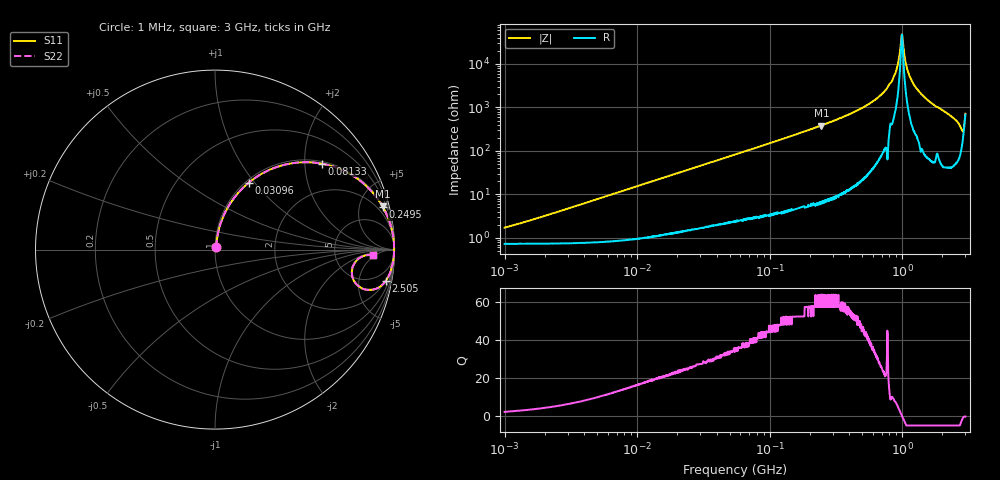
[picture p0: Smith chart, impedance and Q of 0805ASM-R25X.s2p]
!s-Parameter Generated by FASTRON Sdn. Bhd.
!FASTRON P/N : 0805ASM-R25X
!Keysight Technologies: E4991B_MY54100416_A.01.15
!Date: Fri Jun 19 14:51:25 2026
!Version  :Rev00  Fri Jun 19 14:51:25 2026
!Data & Calibration Information:
!Freq  S11  S21  S12  S22
!PortZ  Port1:50+j0  Port2:50+j0
!When reading reference impedance value at option line is always used.
! Remarks : This data is being provided solely for informational purposes.
# Hz S dB R 50
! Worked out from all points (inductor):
!   1601 points, 1 MHz to 3 GHz, reference 50 ohm
!   read as one part in series: L = 247 nH near 1.412 MHz
!   highest Q = 63.5 at 245.8 MHz (marker M1), where L = 249 nH
!   self-resonance near 992.8 MHz
!   S11 on the Smith chart (normalised r, x): 1 MHz: 1.01, +0.03; 30.96 MHz: 1.03, +0.94; 81.33 MHz: 1.06, +2.44; 249.5 MHz: 1.14, +7.87; 2.505 GHz: 2, -11; 3 GHz: 15, -4
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1000000  -35.40 64.0  -0.06 -0.9  -0.06 -0.9  -35.40 64.0
3804036  -24.60 79.3  -0.08 -3.3  -0.08 -3.3  -24.60 79.3
1.447069e7  -13.40 74.8  -0.30 -12.4  -0.30 -12.4  -13.40 74.8
3.096105e7  -7.56 63.2  -0.98 -24.7  -0.98 -24.7  -7.56 63.2
5.504702e7  -4.03 49.4  -2.39 -38.9  -2.39 -38.9  -4.03 49.4
8.132864e7  -2.33 38.8  -4.06 -49.8  -4.06 -49.8  -2.33 38.8
2.083556e8  -0.44 17.2  -10.60 -71.8  -10.60 -71.8  -0.44 17.2
2.457655e8  -0.32 14.5  -12.00 -74.6  -12.00 -74.6  -0.32 14.5
2.494827e8  -0.31 14.2  -12.20 -74.8  -12.20 -74.8  -0.31 14.2
5.337858e8  -0.05 5.2  -20.80 -83.5  -20.80 -83.5  -0.05 5.2
6.889699e8  -0.03 3.0  -25.70 -84.8  -25.70 -84.8  -0.03 3.0
7.925923e8  -0.02 1.8  -30.30 -84.8  -30.30 -84.8  -0.02 1.8
8.937307e8  -0.02 0.9  -36.20 -81.1  -36.20 -81.1  -0.02 0.9
9.730857e8  -0.02 0.2  -48.20 -57.4  -48.20 -57.4  -0.02 0.2
9.977393e8  -0.02 -0.0  -53.60 7.0  -53.60 7.0  -0.02 -0.0
1.023018e9  -0.02 -0.2  -47.30 60.9  -47.30 60.9  -0.02 -0.2
1.108292e9  -0.02 -0.9  -36.30 80.9  -36.30 80.9  -0.02 -0.9
1.255985e9  -0.03 -1.9  -29.50 83.5  -29.50 83.5  -0.03 -1.9
1.581072e9  -0.05 -4.0  -23.10 83.4  -23.10 83.4  -0.05 -4.0
2.505452e9  -0.29 -10.4  -14.80 74.3  -14.80 74.3  -0.29 -10.4
2.811057e9  -1.28 -14.9  -11.20 53.2  -11.20 53.2  -1.28 -14.9
3e9  -1.09 -2.1  -18.20 15.3  -18.20 15.3  -1.09 -2.1
